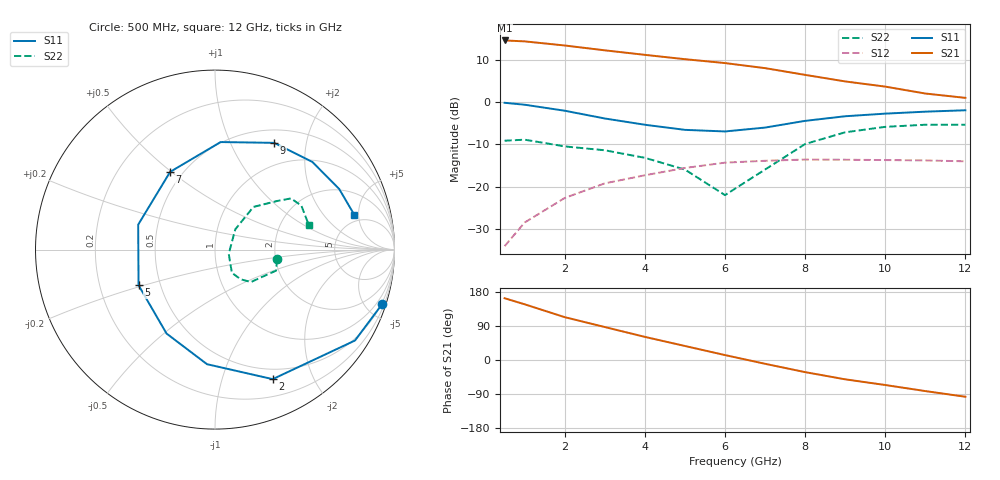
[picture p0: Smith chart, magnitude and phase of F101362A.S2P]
!ATF-10136
!S-PARAMETERS at Vds=2V  Id=25mA.  LAST UPDATED 07-22-92
# ghz s ma r 50
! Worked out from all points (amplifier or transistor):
!   13 points, 500 MHz to 12 GHz, reference 50 ohm
!   highest |S21| = 14.5 dB at 500 MHz (marker M1)
!   |S21| within 3 dB of that: start of sweep to 3.632 GHz
!   unconditionally stable (mu >= 1): 5.298 GHz to end of sweep
!   at 2 GHz: K = 0.67, MSG = 18.0 dB, |S12| = -22.6 dB
!   at 6 GHz: K = 1.02, MAG = 11.0 dB, |S12| = -14.3 dB
!   at 12 GHz: K = 1.06, MAG = 6.0 dB, |S12| = -14.0 dB
!   lowest NFmin = 0.40 dB at 500 MHz
!   S11 on the Smith chart (normalised r, x): 500 MHz: 0.41, -6.29; 2 GHz: 0.38, -1.47; 5 GHz: 0.38, -0.19; 7 GHz: 0.43, +0.49; 9 GHz: 0.67, +1.48; 12 GHz: 4.11, +4.42
0.5  0.98 -18.0  5.32 163.0  0.02 78.0  0.35 -9.0
1  0.93 -33.0  5.19 147.0  0.038 67.0  0.36 -19.0
2  0.79 -66.0  4.64 113.0  0.074 59.0  0.3 -31.0
3  0.64 -94.0  4.07 87.0  0.11 44.0  0.27 -42.0
4  0.54 -120.0  3.6 61.0  0.137 31.0  0.22 -49.0
5  0.47 -155.0  3.2 37.0  0.167 13.0  0.16 -54.0
6  0.45 162.0  2.88 13.0  0.193 -2.0  0.08 -17.0
7  0.5 120.0  2.51 -10.0  0.203 -19.0  0.16 45.0
8  0.6 87.0  2.09 -32.0  0.21 -36.0  0.32 48.0
9  0.68 61.0  1.75 -51.0  0.209 -46.0  0.44 38.0
10  0.73 42.0  1.52 -66.0  0.207 -58.0  0.51 34.0
11  0.77 26.0  1.26 -82.0  0.205 -73.0  0.54 27.0
12  0.8 14.0  1.12 -97.0  0.2 -82.0  0.54 15.0
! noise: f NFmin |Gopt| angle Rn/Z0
0.5  0.4  0.93  12  0.85
1  0.4  0.85  24  0.7
2  0.4  0.7  47  0.46
4  0.5  0.39  126  0.36
6  0.8  0.36  -170  0.12
8  1.1  0.45  -100  0.38
12  1.4  0.6  -41  1.1
